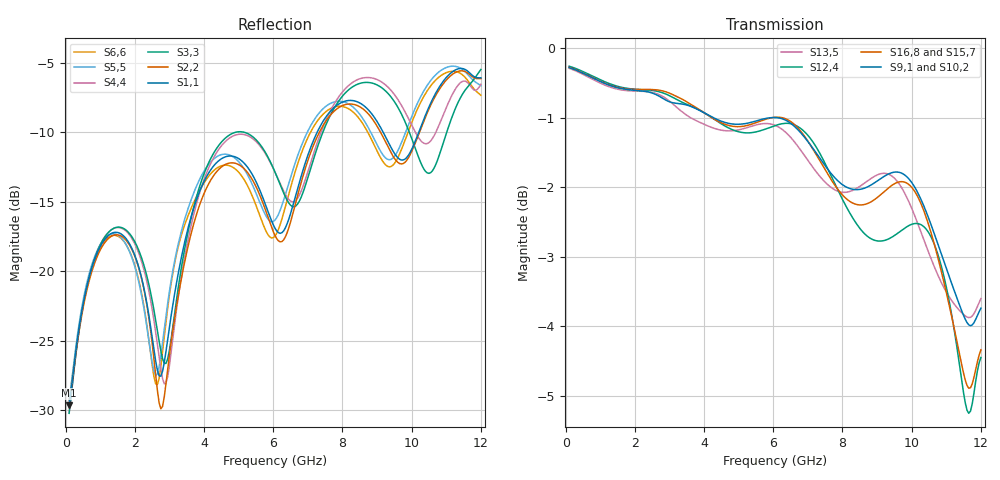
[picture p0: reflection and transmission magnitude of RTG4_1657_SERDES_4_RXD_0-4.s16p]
! RTG4 1657 S-parameter file
! Microsemi Corporation (c) 2019
!Initial ver: Jul 30, 2019
! Port::PIN_NAME::NET_NAME::S-parameter ports::PORT SIDE
! Port1:--:SERDES_4_RXD0_N_DIE::1::DIE
! Port2:--:SERDES_4_RXD0_P_DIE::2::DIE
! Port3:AY29:SERDES_4_RXD0_N_BGA::3::BGA
! Port4:BA29:SERDES_4_RXD0_P_BGA::4::BGA
! Port5:--:SERDES_4_RXD1_N_DIE::5::DIE
! Port6:--:SERDES_4_RXD1_P_DIE::6::DIE
! Port7:AV30:SERDES_4_RXD1_N_BGA::7::BGA
! Port8:AW30:SERDES_4_RXD1_P_BGA::8::BGA
! Port9:--:SERDES_4_RXD2_N_DIE::9::DIE
! Port10:--:SERDES_4_RXD2_P_DIE::10::DIE
! Port11:AY31:SERDES_4_RXD2_N_BGA::11::BGA
! Port12:BA31:SERDES_4_RXD2_P_BGA::12::BGA
! Port13:--:SERDES_4_RXD3_N_DIE::13::DIE
! Port14:--:SERDES_4_RXD3_P_DIE::14::DIE
! Port15:AV32:SERDES_4_RXD3_N_BGA::15::BGA
! Port16:AW32:SERDES_4_RXD3_P_BGA::16::BGA
!TouchstoneFormatFlag = 1
! GNDNET
! NETSLIST
! User Comments:
! Touchstone file exported from HFSS 2018.2.0
!  File:  G:/LSI/Simulation/MASUMIZU/MicroSemi/190627_KD-YB5197_Spara/YBD197_150320_NETCHANGE_SERDES_4_RXD.aedt
!  Generated:  2:24:17 ??  7 10, 2019
!  Design:  HFSSModel1
!  Project:  YBD197_150320_NETCHANGE_SERDES_4_RXD
!  Setup:  Setup1
!  Solution:  Sweep
! Terminal data exported
! Port[1] = SERDES_4_RXD0_N_DIE
! Port[2] = SERDES_4_RXD0_P_DIE
! Port[3] = SERDES_4_RXD1_N_DIE
! Port[4] = SERDES_4_RXD1_P_DIE
! Port[5] = SERDES_4_RXD2_N_DIE
! Port[6] = SERDES_4_RXD2_P_DIE
! Port[7] = SERDES_4_RXD3_N_DIE
! Port[8] = SERDES_4_RXD3_P_DIE
! Port[9] = SERDES_4_RXD0_N_BGA
! Port[10] = SERDES_4_RXD0_P_BGA
! Port[11] = SERDES_4_RXD1_N_BGA
! Port[12] = SERDES_4_RXD1_P_BGA
! Port[13] = SERDES_4_RXD2_N_BGA
! Port[14] = SERDES_4_RXD2_P_BGA
! Port[15] = SERDES_4_RXD3_N_BGA
! Port[16] = SERDES_4_RXD3_P_BGA
# GHZ S DB R 50.000000
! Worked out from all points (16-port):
!   239 points, 100 MHz to 12 GHz, reference 50 ohm
!   strongest paths, dB at 100 MHz, 3.05 GHz, 6.05 GHz, 9.05 GHz, 12 GHz:
!     S9,1: -0.3, -0.8, -1.0, -1.9, -3.7
!     S16,8: -0.3, -0.7, -1.0, -2.1, -4.3
!     S10,2: -0.3, -0.8, -1.1, -2.1, -4.0
!     S15,7: -0.3, -0.6, -1.0, -2.3, -4.2
!     S12,4: -0.3, -0.7, -1.1, -2.8, -4.4
!     S13,5: -0.3, -0.8, -1.1, -1.8, -3.6
!   lowest |S11| = -29.6 dB at 100 MHz (marker M1), VSWR 1.07, Z = 52.9 - j1.75 ohm
!   |S11| at or under -10 dB: start of sweep to 7.268 GHz; 9.176 GHz to 10.2 GHz (1.029 GHz wide, 10.6 % of centre)
